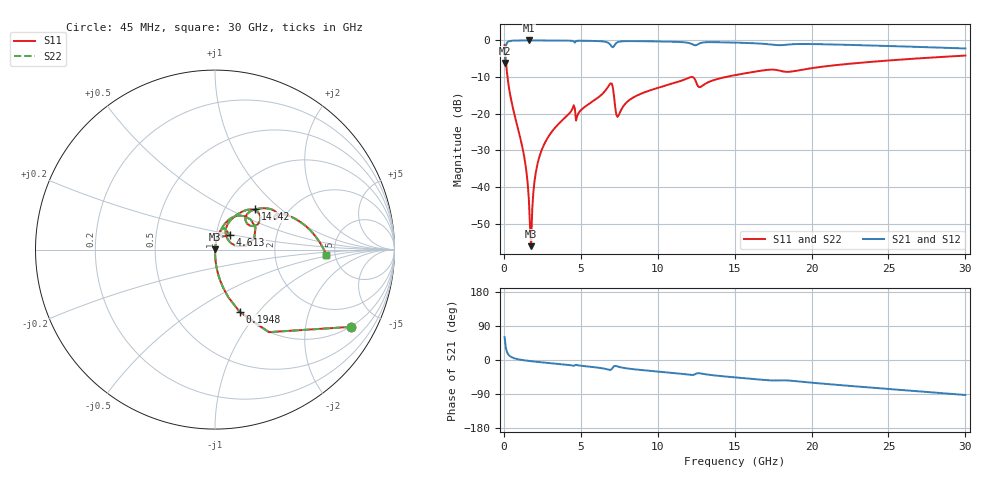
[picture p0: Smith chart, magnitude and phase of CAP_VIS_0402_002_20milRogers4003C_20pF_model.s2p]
! S-parameter model data by Modelithics Inc.  support@modelithics.com  813-866-6335  Tampa FL USA
! S-Parameter data specifications:
! Substrate: 20-mil Rogers 4003C, substrate thickness, H=0.508mm, Dielectric constant, Er=3.75
! PCB Mounting Pad Footprint: Pad width, PadW=0.50mm , Pad length, PadL=0.50mm , Pad gap, PadG (edge-to-edge)=0.40mm , Reference planes=1.4mm apart
! Created Wed Nov 18 12:52:36 2015
# hz S ma R 50
! 2 Port Network Data from SP1.SP block
! freq  magS11  angS11  magS21  angS21  magS12  angS12  magS22  angS22
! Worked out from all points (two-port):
!   401 points, 45 MHz to 30 GHz, reference 50 ohm
!   highest |S21| = -0.01 dB at 1.618 GHz (marker M1); lowest = -6.1 dB at 45 MHz (marker M2)
!   |S21| within 3 dB of the highest: 96.12 MHz to end of sweep
!   lowest |S11| = -56.1 dB at 1.767 GHz (marker M3), VSWR 1.00, Z = 50.1 + j0.104 ohm
!   |S11| at or under -10 dB: 235.5 MHz to 12.16 GHz (11.93 GHz wide, 192 % of centre); 12.27 GHz to 14.4 GHz (2.13 GHz wide, 16 % of centre)
!   |S22| runs from -56.1 to -1.2 dB; largest |S21 - S12| = 0
!   S11 on the Smith chart (normalised r, x): 45 MHz: 1.00, -3.51; 194.8 MHz: 1.00, -0.80; 4.613 GHz: 1.17, +0.19; 14.42 GHz: 1.38, +0.69; 30 GHz: 4.24, -0.42
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4.5e7  0.8693 -29.7  0.4942 60.3  0.4942 60.3  0.8693 -29.7
1.94775e8  0.3726 -68.4  0.9276 21.5  0.9276 21.5  0.3726 -68.4
4.194375e8  0.1752 -80.5  0.984 9.4  0.984 9.4  0.1752 -80.5
1.318088e9  0.02595 -88.7  0.9987 -0.8  0.9987 -0.8  0.02595 -88.7
1.467862e9  0.01593 -88.0  0.9988 -1.7  0.9988 -1.7  0.01593 -88.0
1.617638e9  0.007067 -83.7  0.9989 -2.4  0.9989 -2.4  0.007067 -83.7
1.767412e9  0.001565 41.4  0.9988 -3.1  0.9988 -3.1  0.001565 41.4
1.8423e9  0.005023 73.4  0.9988 -3.5  0.9988 -3.5  0.005023 73.4
2.14185e9  0.01888 81.4  0.9985 -4.8  0.9985 -4.8  0.01888 81.4
2.516288e9  0.03441 81.4  0.998 -6.4  0.998 -6.4  0.03441 81.4
3.414938e9  0.06778 78.8  0.9959 -9.8  0.9959 -9.8  0.06778 78.8
4.613138e9  0.1165 43.2  0.9314 -13.6  0.9314 -13.6  0.1165 43.2
5.062462e9  0.115 73.0  0.9901 -15.4  0.9901 -15.4  0.115 73.0
6.859762e9  0.2491 48.2  0.902 -25.8  0.902 -25.8  0.2491 48.2
7.458862e9  0.09533 47.4  0.9563 -18.0  0.9563 -18.0  0.09533 47.4
8.282625e9  0.1606 63.4  0.9786 -23.7  0.9786 -23.7  0.1606 63.4
1.007992e10  0.2278 58.0  0.9686 -30.7  0.9686 -30.7  0.2278 58.0
1.44234e10  0.3171 45.0  0.9404 -43.7  0.9404 -43.7  0.3171 45.0
1.50225e10  0.3361 42.8  0.9338 -45.9  0.9338 -45.9  0.3361 42.8
2.003996e10  0.42 28.0  0.8924 -60.0  0.8924 -60.0  0.42 28.0
2.505742e10  0.5336 12.7  0.8387 -76.6  0.8387 -76.6  0.5336 12.7
3e10  0.6214 -2.8  0.7767 -92.3  0.7767 -92.3  0.6214 -2.8
